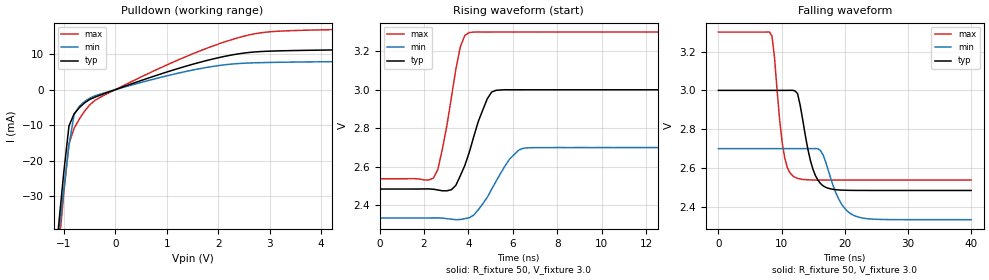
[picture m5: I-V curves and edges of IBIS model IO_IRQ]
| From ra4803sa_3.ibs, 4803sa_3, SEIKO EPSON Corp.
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[Model]   IO_IRQ
Model_type Open_drain
Enable Active-Low
Polarity Non-Inverting
C_comp   5p   4p   6p
[Temperature Range] 25   85   -40
[Voltage Range]   3.0   2.7   3.3
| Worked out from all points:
|   slope of the pulldown table from 0 to 0.45 V, typ, clamps not added: 194 ohm
|   falling waveform, R_fixture 50, V_fixture 3.0: 20-80 % time 1.95ns typ, 2.63ns min, 1.37ns max; typ from 3 V to 2.48 V
|   rising waveform, R_fixture 50, V_fixture 3.0: 20-80 % time 888ps typ, 1.14ns min, 682ps max; typ from 2.48 V to 3 V
[Pulldown]
-3V       -338.5mA   -292.4mA   -359.2mA
-1.1V     -38.27mA   -40.67mA   -44.98mA
-1V       -23.27mA   -28.15mA   -29.11mA
-900mV    -10.27mA   -15.75mA   -15.24mA
-800mV    -6.813mA   -7.063mA   -10.91mA
-700mV    -5.096mA   -4.704mA   -8.327mA
-500mV    -2.786mA   -2.423mA   -4.352mA
-400mV    -2.127mA   -1.753mA   -3.064mA
1.3V      6.319mA    4.911mA    8.886mA
2.6V      10.51mA    7.531mA    15.45mA
3.3V      11mA       7.754mA    16.59mA
6V        11.53mA    8.163mA    17.43mA
[Falling Waveform]
R_fixture=50
V_fixture=3.0
V_fixture_min=2.7
V_fixture_max=3.3
0s        3V         2.7V       3.3V
8.485ns   3V         2.7V       3.279V
10.1ns    3V         2.7V       2.73V
10.91ns   3V         2.7V       2.603V
12.12ns   2.997V     2.7V       2.552V
14.95ns   2.595V     2.7V       2.539V
16.97ns   2.501V     2.633V     2.538V
19.39ns   2.487V     2.42V      2.538V
21.82ns   2.485V     2.351V     2.538V
40ns      2.485V     2.334V     2.538V
[Rising Waveform]
R_fixture=50
V_fixture=3.0
V_fixture_min=2.7
V_fixture_max=3.3
0s        2.485V     2.334V     2.538V
2.424ns   2.484V     2.335V     2.541V
2.828ns   2.475V     2.334V     2.693V
3.636ns   2.554V     2.326V     3.223V
4.04ns    2.676V     2.336V     3.297V
4.444ns   2.835V     2.377V     3.3V
5.051ns   2.989V     2.484V     3.3V
5.859ns   3V         2.641V     3.3V
6.465ns   3V         2.696V     3.3V
20ns      3V         2.7V       3.3V
[Ramp]
R_load=50
dV/dt_r   3.092E-1/8.881E-10   2.195E-1/1.121E-9   4.571E-1/6.661E-10
dV/dt_f   3.085E-1/1.925E-9   1.851E-1/1.941E-9   4.571E-1/1.378E-9
|[End   IO_IRQ
